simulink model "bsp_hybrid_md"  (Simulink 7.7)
settings: Solver=ode45  SolverMode=SingleTasking  StartTime=0.0  StopTime=10.0  FixedStep=0.5  MaxStep=0.01  RelTol=1e-3
undefined symbols (not defined in the file or in its folder): dend, numd, zoh

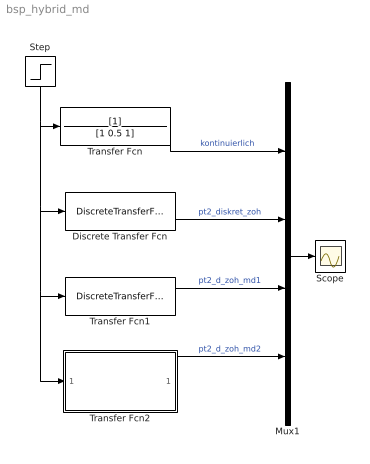
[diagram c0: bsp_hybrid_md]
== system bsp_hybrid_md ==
  Discrete Transfer Fcn : DiscreteTransferFcn  Numerator=[0.1129 0.1038]  Denominator=[1 -1.562 0.7788]  SampleTime=0.5
  Mux1 : Mux
  Scope : Scope
  Step : Step  SampleTime=0
  Transfer Fcn : TransferFcn  Denominator=[1 0.5 1]
  Transfer Fcn1 : DiscreteTransferFcn  Numerator=[0.000000000000000 0.112863280557175 0.103770587465508 ]  Denominator=[1.000000000000000 -1.562166915048721 0.778800783071405 ]  SampleTime=0.5
  Transfer Fcn2 : Subsystem  mask(DiscretizedTransferFcn){Numerator=[1], Denominator=[1 0.5 1], AbsTol=auto, SampleTime=0.5, method=zoh, Wc=0}
      mask prompts: Numerator "Numerator (enter in s-domain:)"; Denominator "Denominator (enter in s-domain:)"; AbsTol "Absolute tolerance:"; SampleTime "Sample time:"; Wc "Critical Frequency (Hz):"
      mask help: Continuous mask uses c2d to transform parameters onto the Discrete Transfer function block inside.
      mask init:
      | st=SampleTime;
      | if length(st)>1
      |     st=SampleTime(1);
      | end
      | if(st>0)
      |     [numd,dend] = sldiscutil('disctransferfcn',{st,method,Wc,Numerator,Denominator});
      | end	
      | s = get_param(gcb,'maskvalues');
      | nums = s{1};
      | dens = s{2};
      | %numc = eval(nums);
      | %denc = eval(dens);
      | sldiscutil('inittfmask', st);
      | if(st==0)
      | set_param([gcb '/Transfer Fcn'], 'AbsoluteTolerance', AbsTol);
      | end
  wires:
  Mux1/1 -> Scope/1
  Transfer Fcn1/1 -> Mux1/3  "pt2_d_zoh_md1"
  Transfer Fcn2/1(Out1) -> Mux1/4  "pt2_d_zoh_md2"
  Transfer Fcn/1 -> Mux1/1  "kontinuierlich"
  Discrete Transfer Fcn/1 -> Mux1/2  "pt2_diskret_zoh"
  Step/1 -> Transfer Fcn/1, Discrete Transfer Fcn/1, Transfer Fcn1/1, Transfer Fcn2/1(In1)

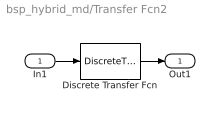
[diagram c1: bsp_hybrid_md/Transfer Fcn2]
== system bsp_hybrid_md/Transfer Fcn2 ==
  In1 : Inport
  Discrete Transfer Fcn : DiscreteTransferFcn  Numerator=numd  Denominator=dend  SampleTime=SampleTime
  Out1 : Outport
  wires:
  In1/1 -> Discrete Transfer Fcn/1
  Discrete Transfer Fcn/1 -> Out1/1
